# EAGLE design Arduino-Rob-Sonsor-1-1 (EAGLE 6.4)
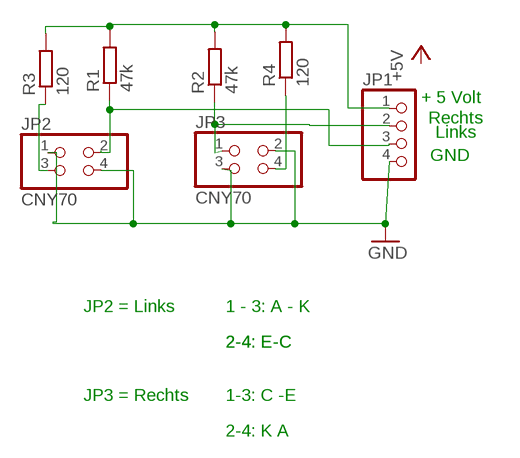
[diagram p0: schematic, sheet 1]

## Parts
JP1  PINHD-1X4  [1X04]
JP2  CNY70  PINHD-2X2  [2X02]
JP3  CNY70  PINHD-2X2  [2X02]
R1  47k  R-10-1  [R-10-1]
R2  47k  R-10-1  [R-10-1]
R3  120  R-10-1  [R-10-1]
R4  120  R-10-1  [R-10-1]

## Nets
CNY70: JP2.3 R3.P$1
GND: JP1.4 JP2.1 JP2.4 JP3.2 JP3.3
N$4: JP3.4 R4.P$1
N$5: JP1.2 JP3.1 R2.P$1
N$7: JP1.3 JP2.2 R1.P$1
N$8: JP1.1 R1.P$2 R2.P$2 R3.P$2 R4.P$2

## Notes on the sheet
- + 5 Volt
- Rechts
- Links
- GND
- JP2 = Links | 1 - 3: A - K
- 2-4: E-C | 2-4: E-C
- JP3 = Rechts | 1-3: C -E
- 2-4: K A

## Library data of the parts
JP1 = pinhead:PINHD-1X4: PIN HEADER
JP2 JP3 = pinhead:PINHD-2X2: PIN HEADER
R1-R4 = papa:R-10-1

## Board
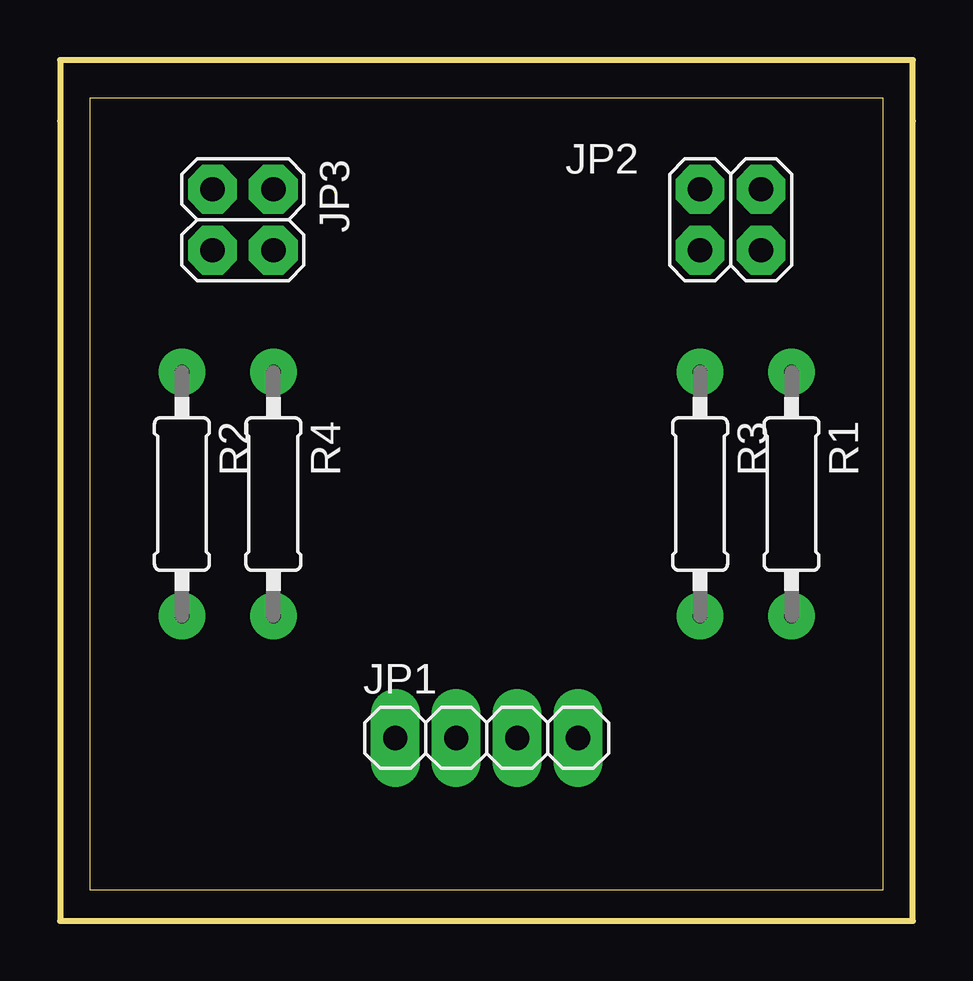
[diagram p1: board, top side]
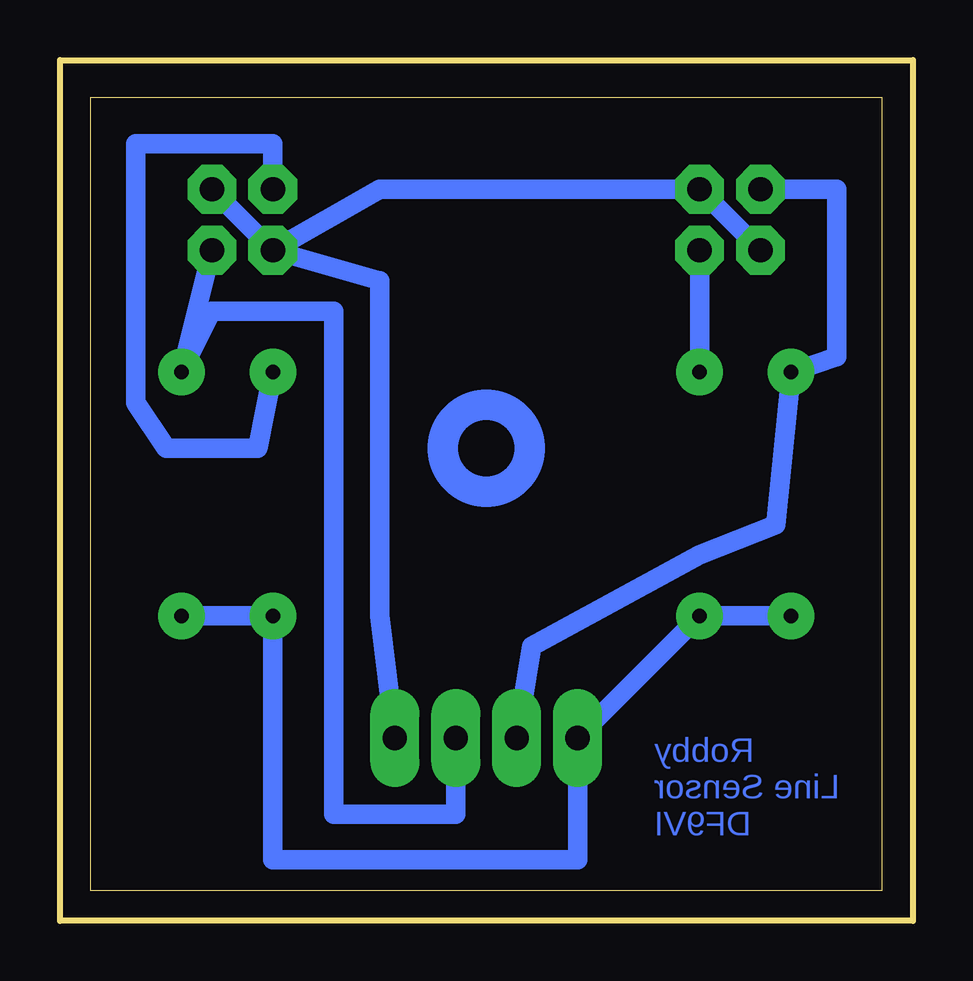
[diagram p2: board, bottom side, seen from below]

Size 35.54 x 35.86 mm. Coordinates in mm from the lower left corner, seen from the top.
Outline: 0,0 35.54,0 35.54,33.32 35.54,35.86 0,35.86 0,33.32 0,0
Outline: 1.27,1.27 1.27,34.29 34.29,34.29 34.29,1.27 1.27,1.27
Copper layers (1*16): Top 0.035mm / dielectric 1.5mm / Bottom 0.035mm
Design rules "default *": minimum track width 30mil, minimum drill 24mil, track to track 8mil, track to pad 8mil, pad to pad 8mil, via to via 8mil, smd to smd 8mil, copper to edge 35mil, drill to drill 8mil, minimum pad ring 20mil, minimum via ring 20mil, stop-mask expansion 4mil, vias tented up to drill 0mil, thermal gap 10mil

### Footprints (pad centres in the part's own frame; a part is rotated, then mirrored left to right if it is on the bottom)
1X04 = drill 1.016 long: 1 -3.81,0; 2 -1.27,0; 3 1.27,0; 4 3.81,0
2X02 = drill 1.016 octagon: 1 -1.27,-1.27; 2 -1.27,1.27; 3 1.27,-1.27; 4 1.27,1.27
R-10-1 = drill 0.6 pad 1.93: P$1 -5.08,0; P$2 5.08,0

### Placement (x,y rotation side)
JP1  17.78,7.62 0 top
JP2  27.94,29.21 180 top
JP3  7.62,29.21 270 top
R1  30.48,17.78 270 top
R2  5.08,17.78 270 top
R3  26.67,17.78 270 top
R4  8.89,17.78 270 top

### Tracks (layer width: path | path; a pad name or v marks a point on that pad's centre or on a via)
CNY70
  Bottom 0.813: R3.P$1 27.3,19.68 31.12,19.68 32.38,21.59 32.38,32.38 26.67,32.38 JP2.3
GND
  Bottom 0.813: JP3.3 JP3.2 22.23,30.48 JP2.4 | JP2.1 JP2.4 | JP1.4 22.23,12.7 22.23,19.05 22.23,26.67 JP2.4
N$4
  Bottom 0.813: R4.P$1 JP3.4
N$5
  Bottom 0.813: JP1.2 15.88,11.43 8.89,15.24 5.71,16.51 R2.P$1 3.18,23.5 3.18,25.4 3.18,30.48 JP3.1
N$7
  Bottom 0.813: JP2.2 R1.P$1 29.21,25.4 24.13,25.4 24.13,16.51 24.13,4.45 19.05,4.45 JP1.3
N$8
  Bottom 0.813: R2.P$2 R4.P$2 JP1.1 13.97,2.54 23.49,2.54 26.67,2.54 26.67,8.89 R3.P$2 R1.P$2
(copper drawn outside any net)
  shapes: Bottom circle x1

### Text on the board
Bottom: Robby / Line Sensor / DF9VI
